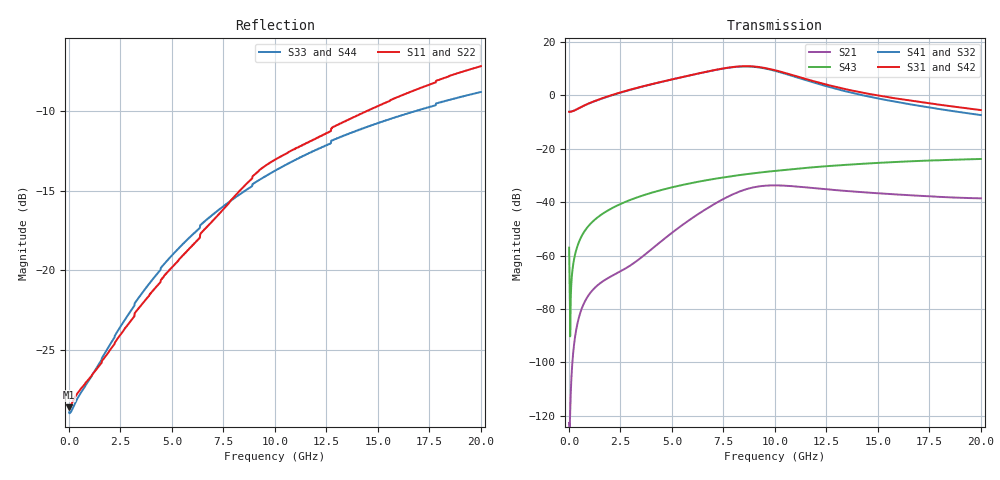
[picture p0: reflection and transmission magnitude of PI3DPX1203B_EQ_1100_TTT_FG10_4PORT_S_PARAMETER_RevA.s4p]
! NPort=4 DATA=2000 NOISE=0 GROUPDELAY=0 COMPLEX_DATAFORMAT=POLAR
! NumOfBlock=1 NumOfParam=0
! .MODEL Smodel S TSTONEFILE=PI3DPX1203B_EQ_1100_TTT_FG10_4PORT_S_PARAMETER_RevA.s4p TYPE=S
!  -- The above .MODEL line can be used for the S element in the netlist.
! The s parameter is extracted from the linear redriver, it is not bi-directional; only s(4,1)s(4,2) and s(3,1)s(3,2)
! should be the insertion loss
!Port definition:
!Port1 = input+
!Port2 = input-
!Port3 = output+
!Port4 = output-
# Hz S MA R  50
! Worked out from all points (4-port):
!   2000 points, 10 MHz to 20 GHz, reference 50 ohm
!   strongest paths, dB at 10 MHz, 5.01 GHz, 10.01 GHz, 15.01 GHz, 20 GHz:
!     S31: -6.2, 6.0, 9.4, -0.1, -5.5
!     S42: -6.2, 6.0, 9.4, -0.1, -5.5
!     S41: -6.2, 6.0, 9.2, -1.2, -7.4
!     S32: -6.2, 6.0, 9.2, -1.2, -7.4
!     S43: -57.1, -34.4, -28.3, -25.3, -23.8
!     S21: -122.7, -51.4, -33.7, -36.7, -38.6
!   lowest |S11| = -28.6 dB at 10 MHz (marker M1), VSWR 1.08, Z = 46.4 - j0.0306 ohm
!   |S11| at or under -10 dB: start of sweep to 14.43 GHz
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1e7  0.03701 -179.5  7.338e-07 10.7  0 0.0  0 0.0
     7.338e-07 10.7  0.03701 -179.5  0 0.0  0 0.0
     0.4917 0.0  0.4917 -180.0  0.03566 178.2  0.001403 -77.8
     0.4917 -180.0  0.4917 0.0  0.001403 -77.8  0.03566 178.2
3.08e9  0.07025 -126.9  0.0006923 142.6  1.452e-10 55.7  2.594e-09 107.3
        0.0006921 142.6  0.07025 -126.9  2.594e-09 107.3  1.452e-10 55.7
        1.31 2.6  1.298 -176.2  0.07565 -126.7  0.01139 77.7
        1.298 -176.2  1.31 2.6  0.01139 77.7  0.07565 -126.7
5.78e9  0.1157 -111.0  0.004433 154.3  1.179e-08 -122.1  1.08e-07 69.6
        0.004433 154.4  0.1157 -111.0  1.08e-07 69.6  1.18e-08 -122.1
        2.322 -39.2  2.32 142.2  0.1254 -117.3  0.02208 66.2
        2.321 142.2  2.322 -39.2  0.02208 66.2  0.1254 -117.3
8.17e9  0.1743 -104.9  0.01519 111.0  2.988e-07 155.6  8.356e-07 20.4
        0.01519 111.0  0.1743 -104.9  8.348e-07 20.4  2.989e-07 155.6
        3.455 -98.7  3.423 82.5  0.171 -115.8  0.03167 54.0
        3.424 82.5  3.454 -98.7  0.03167 54.0  0.171 -115.8
9.72e9  0.2168 -107.2  0.02054 67.3  1.044e-06 94.7  1.771e-06 -17.2
        0.02052 67.4  0.2168 -107.2  1.769e-06 -17.1  1.045e-06 94.7
        3.134 -148.9  3.061 32.2  0.2004 -116.2  0.03748 45.9
        3.063 32.2  3.133 -148.9  0.03748 45.9  0.2004 -116.2
1.195e10  0.2587 -109.3  0.01826 26.3  2.818e-06 29.7  3.494e-06 -45.5
          0.01824 26.4  0.2587 -109.3  3.494e-06 -45.4  2.82e-06 29.7
          1.808 162.7  1.703 -16.1  0.2387 -117.4  0.04529 34.4
          1.704 -16.1  1.807 162.7  0.04529 34.4  0.2387 -117.4
2e10  0.4387 -117.6  0.01172 -17.7  2.239e-05 -109.4  3.126e-05 -133.8
      0.01178 -17.5  0.4388 -117.7  3.134e-05 -133.7  2.242e-05 -109.4
      0.5294 74.2  0.4268 -93.4  0.3637 -123.9  0.06431 -7.1
      0.4266 -93.6  0.5299 74.3  0.06431 -7.1  0.3637 -123.9
